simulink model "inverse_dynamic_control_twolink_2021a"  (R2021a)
settings: Solver=VariableStepAuto  StartTime=0.0  StopTime=maxtime  RelTol=1e-3
InitFcn:
  | stop_time_as_str = get_param(gcs, 'StopTime');
  | stopTime = str2double(stop_time_as_str);
undefined symbols (not defined in the file or in its folder): KD, KP, max_torques, min_torques
libraries: roblocks x3

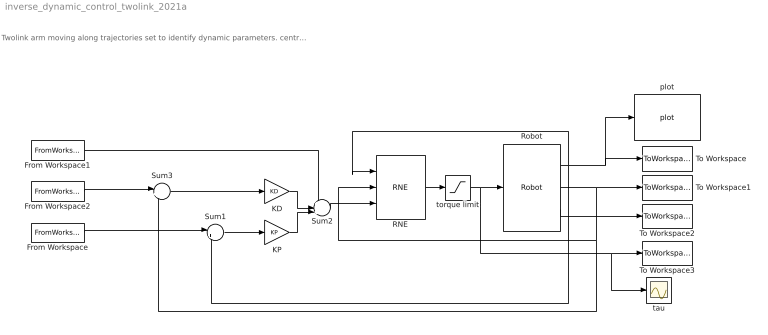
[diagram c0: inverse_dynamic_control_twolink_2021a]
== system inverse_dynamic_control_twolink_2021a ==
  note: Twolink arm moving along trajectories set to identify dynamic parameters. centralized_control_design_twolink.m should be run first.
  From Workspace : FromWorkspace  VariableName=qT
  From Workspace1 : FromWorkspace  VariableName=qddT
  From Workspace2 : FromWorkspace  VariableName=qdT
  KD : Gain  Gain=KD
  KP : Gain  Gain=KP
  RNE : roblocks/Arm/RNE  robot=twolink  grav=[0 9.81 0]
  Robot : roblocks/Arm/Robot  robot=twolink  q0=q0
  Sum1 : Sum  Inputs=|+-
  Sum2 : Sum  Inputs=+++|
  Sum3 : Sum  Inputs=|+-
  To Workspace : ToWorkspace  VariableName=qout  SampleTime=-1
  To Workspace1 : ToWorkspace  VariableName=qdout  SampleTime=-1
  To Workspace2 : ToWorkspace  VariableName=qddout  SampleTime=-1
  To Workspace3 : ToWorkspace  VariableName=Qout  SampleTime=-1
  plot : roblocks/Arm/plot  robot=twolink  fps=10  holdplot=on
  tau : Scope
  torque limit : Saturate  UpperLimit=max_torques  LowerLimit=min_torques
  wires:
  Robot/3 -> To Workspace2/1
  Sum1/1 -> KP/1
  From Workspace/1 -> Sum1/1
  RNE/1 -> torque limit/1
  Sum2/1 -> RNE/3
  Robot/1 -> Sum1/2, To Workspace/1, plot/1, RNE/1
  Robot/2 -> Sum3/2, RNE/2, To Workspace1/1
  KP/1 -> Sum2/3
  KD/1 -> Sum2/2
  From Workspace1/1 -> Sum2/1
  Sum3/1 -> KD/1
  From Workspace2/1 -> Sum3/1
  torque limit/1 -> tau/1, To Workspace3/1, Robot/1
